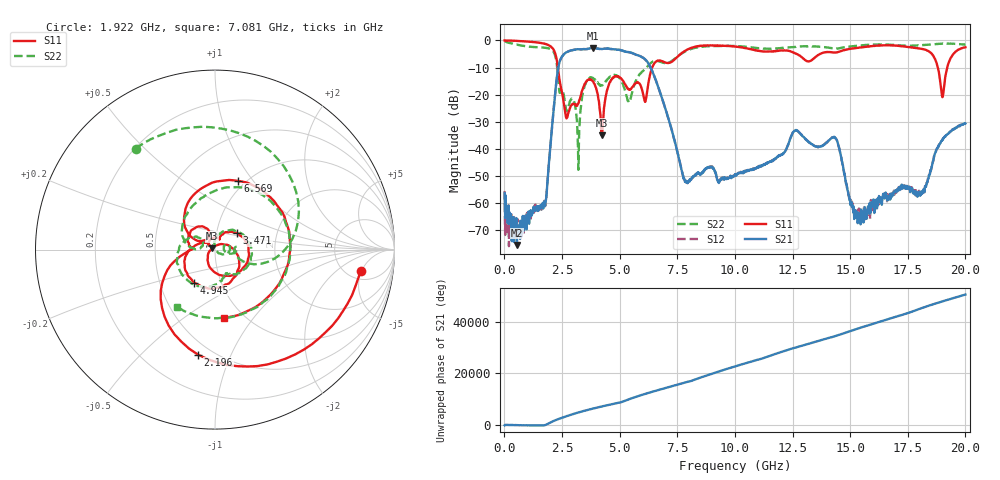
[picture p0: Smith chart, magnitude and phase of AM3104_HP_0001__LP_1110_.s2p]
!Created with skrf (http://scikit-rf.org).
# Hz S RI R 50.0
!freq ReS11 ImS11 ReS21 ImS21 ReS12 ImS12 ReS22 ImS22
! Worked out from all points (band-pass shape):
!   1601 points, 10 MHz to 20 GHz, reference 50 ohm
!   highest |S21| = -2.75 dB at 3.833 GHz (marker M1); lowest = -75.6 dB at 547.2 MHz (marker M2)
!   |S21| within 3 dB of the highest: 2.516 GHz to 5.894 GHz (3.378 GHz wide, 80.3 % of centre)
!   lowest |S11| = -35.1 dB at 4.22 GHz (marker M3), VSWR 1.04, Z = 48.5 + j0.792 ohm
!   |S11| at or under -10 dB: 2.322 GHz to 6.411 GHz (4.089 GHz wide, 93.7 % of centre); 18.8 GHz to 19.21 GHz (408 MHz wide, 2.15 % of centre)
!   |S22| runs from -47.8 to -0.2 dB; largest |S21 - S12| = 0.0076
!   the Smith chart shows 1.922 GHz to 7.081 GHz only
!   S11 on the Smith chart (normalised r, x): 1.922 GHz: 6.64, -4.81; 2.196 GHz: 0.42, -0.76; 3.471 GHz: 1.26, +0.24; 4.945 GHz: 0.74, -0.29; 6.569 GHz: 0.93, +0.84; 7.081 GHz: 0.81, -0.73
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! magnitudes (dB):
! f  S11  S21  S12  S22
! 10 MHz  0.0  -56.4  -55.6  -0.2
! 547.2 MHz  -0.1  -75.6  -68.3  -1.5
! 1.922 GHz  -1.7  -46.7  -46.5  -2.9
! 2.196 GHz  -4.5  -20.2  -20.2  -5.4
! 2.696 GHz  -28.8  -4.4  -4.3  -26.1
! 3.346 GHz  -19.3  -3.3  -3.2  -22.5
! 3.471 GHz  -16.2  -3.2  -3.2  -17.1
! 3.833 GHz  -14.9  -2.8  -2.7  -13.8
! 4.22 GHz  -35.1  -3.1  -3.1  -16.6
! 4.945 GHz  -13.2  -3.4  -3.4  -13.5
! 6.569 GHz  -7.9  -14.6  -14.6  -7.5
! 6.682 GHz  -7.4  -17.4  -17.4  -7.7
! 7.081 GHz  -8.3  -27.9  -27.9  -8.3
! 7.869 GHz  -3.7  -52.4  -52.3  -3.9
! 10.01 GHz  -2.2  -49.4  -49.7  -2.1
! 13.34 GHz  -7.2  -38.3  -38.3  -2.2
! 14.38 GHz  -4.4  -36.2  -36.3  -3.0
! 15.35 GHz  -2.7  -64.9  -63.8  -1.9
! 16.68 GHz  -1.8  -58.1  -57.6  -1.6
! 18.1 GHz  -3.1  -56.7  -56.4  -1.7
! 19 GHz  -20.9  -36.6  -36.6  -1.2
! 20 GHz  -2.5  -30.7  -30.7  -1.5
